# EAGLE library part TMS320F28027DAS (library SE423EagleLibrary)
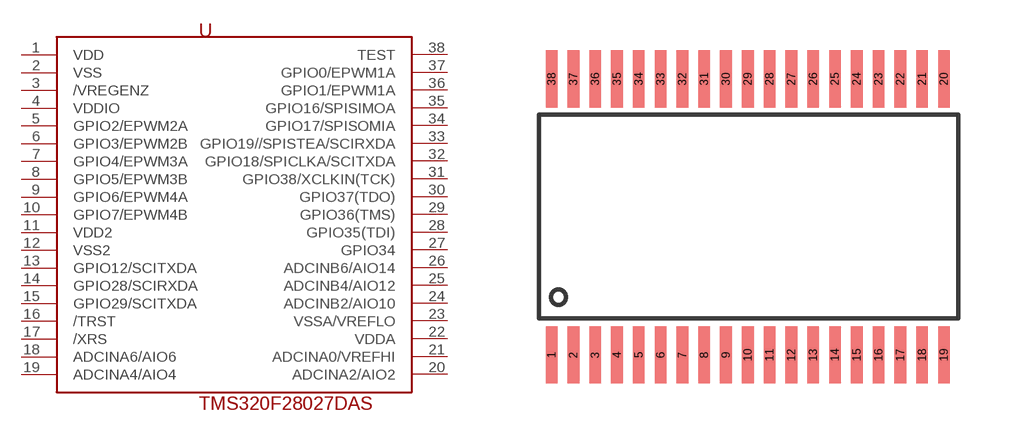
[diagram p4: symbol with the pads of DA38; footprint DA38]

Designator prefix U

## TMS320F28027DAS  [DA38]
1  VDD
2  VSS
3  /VREGENZ
4  VDDIO
5  GPIO2/EPWM2A
6  GPIO3/EPWM2B
7  GPIO4/EPWM3A
8  GPIO5/EPWM3B
9  GPIO6/EPWM4A
10  GPIO7/EPWM4B
11  VDD2
12  VSS2
13  GPIO12/SCITXDA
14  GPIO28/SCIRXDA
15  GPIO29/SCITXDA
16  /TRST
17  /XRS
18  ADCINA6/AIO6
19  ADCINA4/AIO4
20  ADCINA2/AIO2
21  ADCINA0/VREFHI
22  VDDA
23  VSSA/VREFLO
24  ADCINB2/AIO10
25  ADCINB4/AIO12
26  ADCINB6/AIO14
27  GPIO34
28  GPIO35(TDI)
29  GPIO36(TMS)
30  GPIO37(TDO)
31  GPIO38/XCLKIN(TCK)
32  GPIO18/SPICLKA/SCITXDA
33  GPIO19//SPISTEA/SCIRXDA
34  GPIO17/SPISOMIA
35  GPIO16/SPISIMOA
36  GPIO1/EPWM1A
37  GPIO0/EPWM1A
38  TEST

## Footprint DA38 (pad centres in mm)
smd 0.35 x 1.705: 1 -5.85,-4.12; 2 -5.2,-4.12; 3 -4.55,-4.12; 4 -3.9,-4.12; 5 -3.25,-4.12; 6 -2.6,-4.12; 7 -1.95,-4.12; 8 -1.3,-4.12; 9 -0.65,-4.12; 10 0,-4.12; 11 0.65,-4.12; 12 1.3,-4.12; 13 1.95,-4.12; 14 2.6,-4.12; 15 3.25,-4.12; 16 3.9,-4.12; 17 4.55,-4.12; 18 5.2,-4.12; 19 5.85,-4.12; 20 5.85,4.12; 21 5.2,4.12; 22 4.55,4.12; 23 3.9,4.12; 24 3.25,4.12; 25 2.6,4.12; 26 1.95,4.12; 27 1.3,4.12; 28 0.65,4.12; 29 0,4.12; 30 -0.65,4.12; 31 -1.3,4.12; 32 -1.95,4.12; 33 -2.6,4.12; 34 -3.25,4.12; 35 -3.9,4.12; 36 -4.55,4.12; 37 -5.2,4.12; 38 -5.85,4.12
